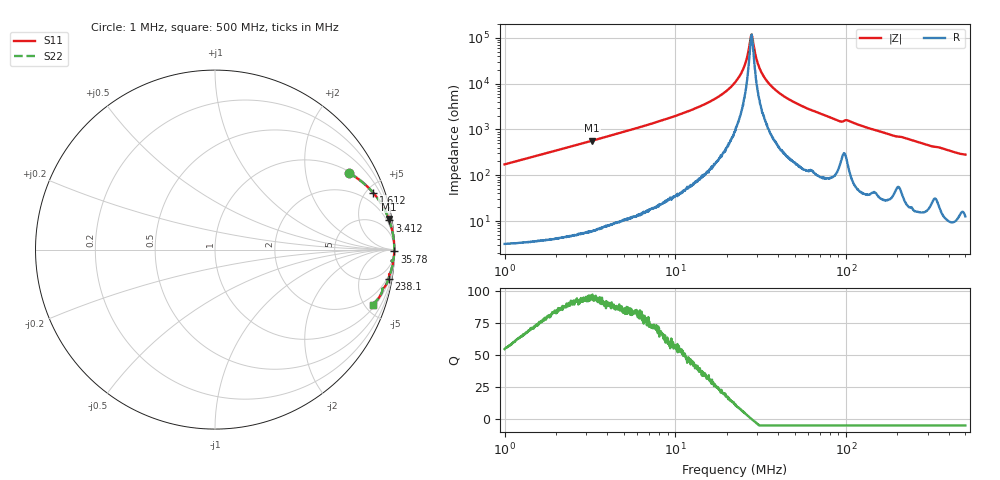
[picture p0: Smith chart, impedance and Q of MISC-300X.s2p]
!s-Parameter Generated by FASTRON Sdn. Bhd.
!FASTRON P/N : MISC-300X
!Keysight Technologies,E4991B,MY54100416,A.01.15
!Date: Thu Mar 26 10:47:37 2026
!Version  : Rev00 Thu Mar 26 10:47:37 2026
!Data & Calibration Information:
!PortZ  Port1:50+j0  Port2:50+j0
!When reading, reference impedance value at option line is always used.
!Remarks : This data is being provided solely for informational purposes.
!Freq	S11	S21	S12	S22
# Hz S dB R 50
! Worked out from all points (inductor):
!   1601 points, 1 MHz to 500 MHz, reference 50 ohm
!   read as one part in series: L = 27.4 uH near 1.032 MHz
!   highest Q = 94.8 at 3.257 MHz (marker M1), where L = 27.8 uH
!   self-resonance near 27.9 MHz
!   S11 on the Smith chart (normalised r, x): 1 MHz: 1.06, +3.45; 1.612 MHz: 1.07, +5.57; 3.412 MHz: 1, +12; 35.78 MHz: open; 238.1 MHz: 1, -12; 500 MHz: 1.25, -5.64
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1000000  -1.33 29.8  -6.06 -59.1  -6.06 -59.1  -1.33 29.8
1612439  -0.56 19.7  -9.46 -69.6  -9.46 -69.6  -0.56 19.7
2820919  -0.20 11.5  -14.01 -77.9  -14.01 -77.9  -0.20 11.5
3256899  -0.15 10.0  -15.24 -79.4  -15.24 -79.4  -0.15 10.0
3412295  -0.14 9.5  -15.64 -79.9  -15.64 -79.9  -0.14 9.5
7957584  -0.03 3.8  -23.47 -85.4  -23.47 -85.4  -0.03 3.8
1.552103e7  -0.01 1.5  -31.73 -86.7  -31.73 -86.7  -0.01 1.5
1.914303e7  -0.01 0.9  -35.79 -86.1  -35.79 -86.1  -0.01 0.9
2.236068e7  -0.01 0.5  -40.52 -84.6  -40.52 -84.6  -0.01 0.5
2.522189e7  -0.01 0.2  -47.20 -78.4  -47.20 -78.4  -0.01 0.2
2.736538e7  -0.01 0.1  -58.10 -46.1  -58.10 -46.1  -0.01 0.1
2.790203e7  -0.01 0.0  -61.13 -7.4  -61.13 -7.4  -0.01 0.0
2.855992e7  -0.01 -0.1  -58.04 46.1  -58.04 46.1  -0.01 -0.1
2.980659e7  -0.01 -0.2  -51.04 71.2  -51.04 71.2  -0.01 -0.2
3.122875e7  -0.01 -0.3  -46.60 79.0  -46.60 79.0  -0.01 -0.3
3.577623e7  -0.01 -0.6  -39.61 84.3  -39.61 84.3  -0.01 -0.6
4.464218e7  -0.01 -1.2  -33.86 85.8  -33.86 85.8  -0.01 -1.2
6.307767e7  -0.02 -2.2  -28.39 85.1  -28.39 85.1  -0.02 -2.2
9.122775e7  -0.08 -3.7  -23.74 80.5  -23.74 80.5  -0.08 -3.7
1.77937e8  -0.11 -7.2  -18.03 80.7  -18.03 80.7  -0.11 -7.2
2.381115e8  -0.17 -9.5  -15.65 78.6  -15.65 78.6  -0.17 -9.5
5e8  -0.63 -19.2  -9.64 68.2  -9.64 68.2  -0.63 -19.2
